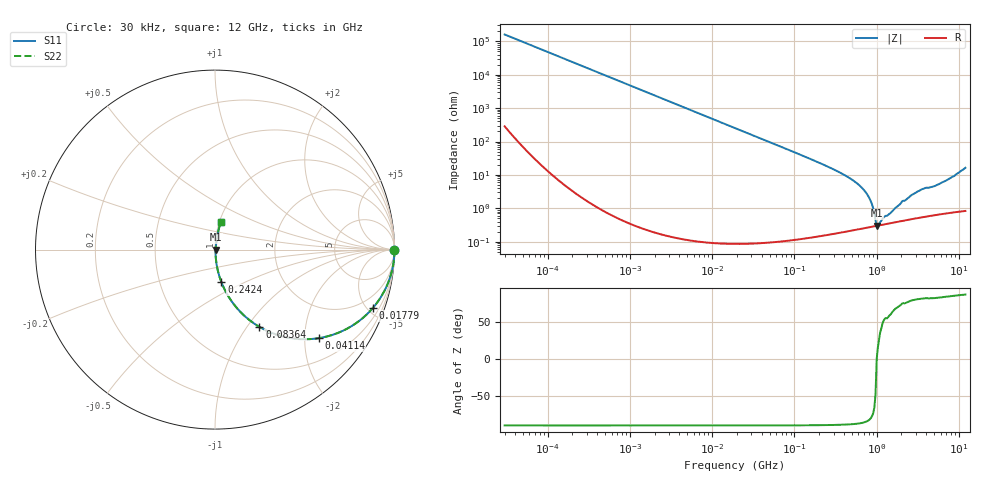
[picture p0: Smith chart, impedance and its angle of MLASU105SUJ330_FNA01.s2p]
! MLASU105SUJ330_FNA01  S-PARAMETER MODEL  ( General Type )
! Model Generated by TAIYO YUDEN Corporation (http://www.ty-top.com)
! Version 4.0
! TAIYO YUDEN Control No. 120810
! Copyright(c) 2003 TAIYO YUDEN CO.,LTD. All Rights Reserved.
! Product Description (link to TY-COMPAS)
! https://ds.yuden.co.jp/TYCOMPAS/or/detail?pn=MLASU105SUJ330JFNA01&u=M
! Products Name : Multilayer Ceramic Capacitors
! Characteristics :
!  Capacitance : 33 pF , Rated Voltage : 50V , TCC : UJ / U2J
!  Case Size : 1.0 x 0.5 / 0.039 x 0.02 [mm/inch] , Thickness : 0.5 / 0.02 [mm/inch]
!  (Conditions: Temperature = 25 degC , DC Bias Current/Voltage = 0A / 0V)
! External Node Assignments :
!  1  o---| |---o  2
! GND o---------o GND
! Frequency Range : 0.03MHz  -  12000MHz  [ 401 STEP ]
# MHz S RI R 50
! Freq[MHz].  S11 Real  S11 Imag  S21 Real  S21 Imag  S12 Real  S12 Imag  S22 Real  S22 Imag
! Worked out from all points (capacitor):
!   401 points, 30 kHz to 12 GHz, reference 50 ohm
!   read as one part in series: C = 33 pF near 32 kHz
!   lowest |Z| = 299 mohm at 1.002 GHz (marker M1)
!   series resonance near 1.002 GHz, so ESL is about 760 pH
!   S11 on the Smith chart (normalised r, x): 30 kHz: open; 17.79 MHz: 1.00, -5.42; 41.14 MHz: 1.00, -2.34; 83.64 MHz: 1.00, -1.15; 242.4 MHz: 1.00, -0.37; 12 GHz: 1.02, +0.33
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0.03  1 -0.000622  1.49e-06 0.000622  1.49e-06 0.000622  1 -0.000622
0.260295  1 -0.0054  2.97e-05 0.0054  2.97e-05 0.0054  1 -0.0054
2.258455  0.9978 -0.0467  0.00219 0.0467  0.00219 0.0467  0.9978 -0.0467
6.982189  0.9794 -0.1418  0.0206 0.1418  0.0206 0.1418  0.9794 -0.1418
17.78857  0.8801 -0.3247  0.1199 0.3247  0.1199 0.3247  0.8801 -0.3247
18.97367  0.8658 -0.3407  0.1342 0.3407  0.1342 0.3407  0.8658 -0.3407
41.141  0.5779 -0.4935  0.4221 0.4935  0.4221 0.4935  0.5779 -0.4935
83.63502  0.2474 -0.4305  0.7526 0.4305  0.7526 0.4305  0.2474 -0.4305
164.6252  0.0762 -0.263  0.9238 0.263  0.9238 0.263  0.0762 -0.263
242.4142  0.0353 -0.1804  0.9647 0.1804  0.9647 0.1804  0.0353 -0.1804
462.0203  0.00875 -0.0814  0.9913 0.0814  0.9913 0.0814  0.00875 -0.0814
680.3351  0.00393 -0.038  0.9961 0.038  0.9961 0.038  0.00393 -0.038
825.5698  0.00307 -0.0187  0.9969 0.0187  0.9969 0.0187  0.00307 -0.0187
880.5704  0.00296 -0.0125  0.997 0.0125  0.997 0.0125  0.00296 -0.0125
1001.808  0.00298 -5.1e-06  0.997 5.1e-06  0.997 5.1e-06  0.00298 -5.1e-06
1068.55  0.00308 0.00147  0.9969 -0.00147  0.9969 -0.00147  0.00308 0.00147
1215.67  0.00329 0.00415  0.9967 -0.00415  0.9967 -0.00415  0.00329 0.00415
1428.372  0.00356 0.00579  0.9964 -0.00579  0.9964 -0.00579  0.00356 0.00579
2811.574  0.00551 0.0262  0.9945 -0.0262  0.9945 -0.0262  0.00551 0.0262
3758.338  0.00691 0.038  0.9931 -0.038  0.9931 -0.038  0.00691 0.038
5534.236  0.00888 0.0498  0.9911 -0.0498  0.9911 -0.0498  0.00888 0.0498
12000  0.0335 0.1563  0.9665 -0.1563  0.9665 -0.1563  0.0335 0.1563
